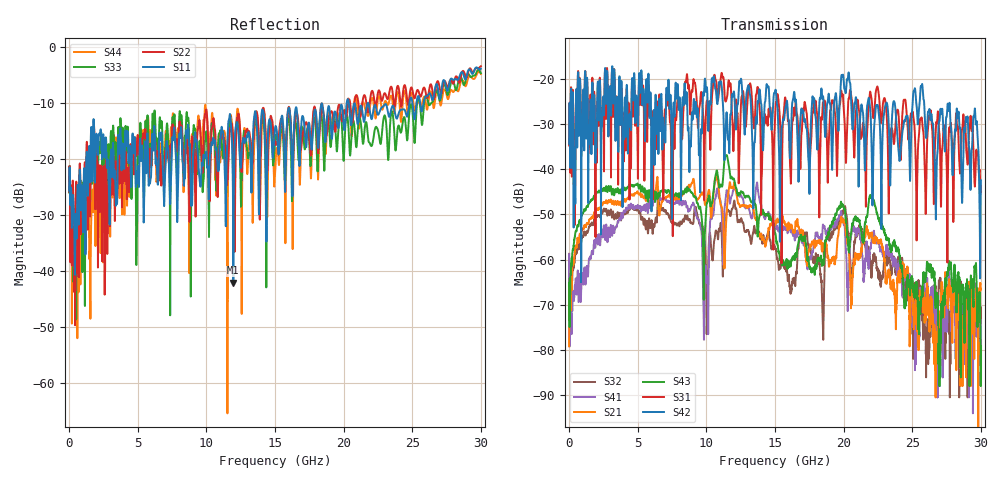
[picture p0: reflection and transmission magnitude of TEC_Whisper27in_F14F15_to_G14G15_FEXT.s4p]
! Tyco Electronics
! F14F15-G14G15_FEXT
!! PART DESCRIPTION: Whisper 27in Megtron 6 VLP-HVLP-VLP Channel Model, bulkhead 2.4mm test pts
!! MODEL DESCRIPTION: System 4-port S-parameter
!! MODEL STATUS: Measured
!! MODEL GEOMETRY: Channel Model
!! MODEL FREQUENCY RANGE: DC to 30.000 GHz in 10.000 MHz frequency steps
!! MODEL EDGE RATE LIMITATION: 12.500 ps (Using conservative 0.5/Fmax rule of thumb)
!! TIME-DOMAIN TRANSFORM CAUTIONS:
!! 1.) Do not simulate transient edge rates faster than the number listed above.  Edge rates faster than this number
!!  contain significant spectral content at frequencies above the model's highest frequency.
!! 2.) Even when simulating edge rates that are slower than the number listed above, be aware that the best time
!!  resolution possible with a direct iFFT is (1 / 2Fmax).  As a result, time resolution is typically not adequate
!!  for most time-domain simulations unless tricks such as windowing are used to minimize leakage and aliasing.
!! 3.) Because the model has a uniform frequency step, a direct iFFT will result in an impulse that that has a time
!!  length given by either (1 / Fstep) or (1 / 2Fstep), depending on the transform being used.  Care has been taken
!!  in selecting the frequency step to ensure a settled impulse response for the model.  Therefore, convolution with
!!  the model's impulse response should present no issues.  However, if directly concatenating s-parameter models
!!  in the frequency domain a user must either interpolate necessary interim frequencies or complete impulse response
!!  zero-padding.  Impulse response zero-padding is more difficult, but more accurate.
!! PORT DEFINITIONS:
!! Port  1  ----->  Side A  F14  G14  Side B  <-----  Port  2
!! Port  3  ----->  Side A  F15  G15  Side B  <-----  Port  4
! Point-to-Point link (differential)  !
! Connectors:  !
!  1: STRADA Whisper  !
! Materials:  !
!  Backplane: Megtron-6 HVLP  !
!  Daughtercard: Megtron-6 VLP  !
! Stack-up:  !
!  Backplane: 20 layers, 200mil thick  !
!  Daughtercard: 14 layers, 110mil thick  !
! Trace Length:  !
!  Backplane: 17in  !
!  Daightercards: 5in  !
! Trace Width:  !
!  Backplane: 8-13-8 mils  !
!  Daughtercards: 6-9-6 mils  !
! Geometry:  !
!  Backplane: Stripline  !
!  Daughtercards: Stripline  !
! Freq. Range: 0 GHz - 30 GHz  !
! Note1: non-mixed-mode s-parameters  !
! Note2: channel includes 2.4mm test points  !
! Touchstone data converted from IdEM dataset
# GHz S MA R 50
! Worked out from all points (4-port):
!   3000 points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, 10 MHz to 30 GHz, reference 50 ohm
!   strongest paths, dB at 10 MHz, 7.51 GHz, 15.01 GHz, 22.51 GHz, 30 GHz:
!     S42: -34.4, -40.9, -22.7, -26.2, -42.5
!     S31: -34.8, -36.1, -28.5, -22.3, -45.0
!     S43: -65.7, -46.1, -54.2, -50.7, -79.2
!     S21: -79.2, -46.6, -52.1, -56.3, -66.6
!     S41: -58.8, -47.6, -52.4, -56.1, -79.2
!     S32: -58.7, -51.9, -57.5, -62.7, -74.0
!   lowest |S11| = -42.0 dB at 11.97 GHz (marker M1), VSWR 1.02, Z = 49.4 - j0.466 ohm
!   |S11| at or under -10 dB: start of sweep to 18.4 GHz; 18.41 GHz to 20.23 GHz (1.812 GHz wide, 9.38 % of centre); 21.81 GHz to 24.79 GHz (2.983 GHz wide, 12.8 % of centre)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
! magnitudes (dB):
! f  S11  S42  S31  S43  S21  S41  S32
! 10 MHz  -25.6  -34.4  -34.8  -65.7  -79.2  -58.8  -58.7
! 2.59 GHz  -19.5  -21.3  -21.8  -44.5  -47.5  -53.5  -49.0
! 9.03 GHz  -20.3  -28.6  -21.1  -45.5  -42.4  -47.4  -52.0
! 9.91 GHz  -19.5  -20.0  -32.0  -53.3  -47.9  -61.9  -56.8
! 11.97 GHz  -42.0  -23.4  -36.0  -42.0  -44.0  -44.6  -48.0
! 25.71 GHz  -11.4  -21.2  -29.0  -66.0  -71.7  -66.9  -69.4
! 30 GHz  -3.8  -42.5  -45.0  -79.2  -66.6  -79.2  -74.0
